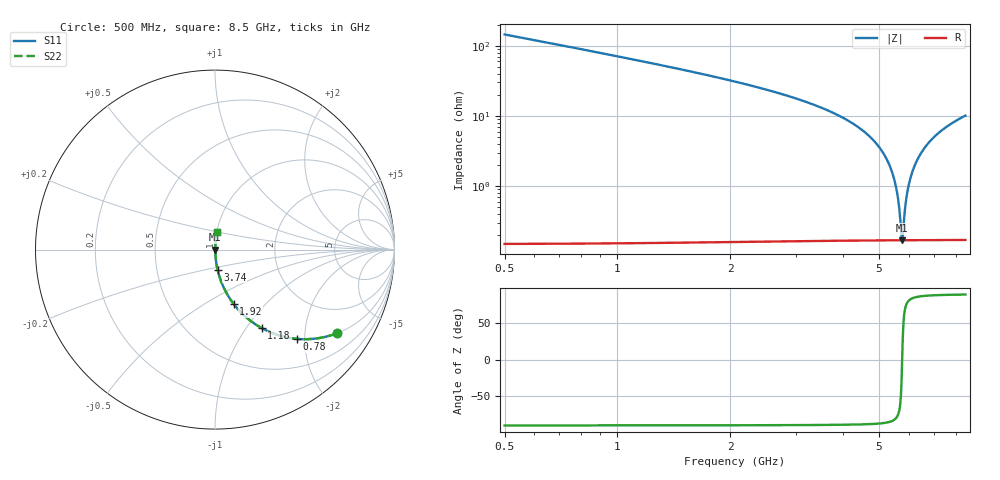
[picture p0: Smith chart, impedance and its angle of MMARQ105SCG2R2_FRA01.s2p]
! MMARQ105SCG2R2_FRA01  S-PARAMETER MODEL  ( General Type )
! Model Generated by TAIYO YUDEN Corporation (http://www.ty-top.com)
! Version 1.0
! TAIYO YUDEN Control No. 200326
! Copyright(c) 2020 TAIYO YUDEN CO.,LTD. All Rights Reserved.
! Product Description (link to TY-COMPAS)
! https://ds.yuden.co.jp/TYCOMPAS/or/detail?pn=MMARQ105SCG2R2BFRA01&u=M
! Products Name : Multilayer Ceramic Capacitors
! Characteristics :
!  Capacitance : 2.2 pF , Rated Voltage : 250V , TCC : CG / C0G
!  Case Size : 1.0 x 0.5 / 0.039 x 0.02 [mm/inch] , Thickness : 0.5 / 0.02 [mm/inch]
!  (Conditions: Temperature = 25 degC , DC Bias Current/Voltage = 0A / 0V)
! External Node Assignments :
!  1  o---| |---o  2
! GND o---------o GND
! Frequency Range : 500MHz  -  8.5GHz  [ 401 STEP ]
# MHz S RI R 50
! Freq[MHz].  S11 Real  S11 Imag  S21 Real  S21 Imag  S12 Real  S12 Imag  S22 Real  S22 Imag
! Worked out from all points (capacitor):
!   401 points, 500 MHz to 8.5 GHz, reference 50 ohm
!   read as one part in series: C = 2.18 pF near 540 MHz
!   lowest |Z| = 169 mohm at 5.76 GHz (marker M1)
!   series resonance near 5.762 GHz, so ESL is about 350 pH
!   S11 on the Smith chart (normalised r, x): 500 MHz: 1.00, -2.90; 780 MHz: 1.00, -1.84; 1.18 GHz: 1.00, -1.19; 1.92 GHz: 1.00, -0.68; 3.74 GHz: 1.00, -0.23; 8.5 GHz: 1.00, +0.20
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500  0.6773 -0.467  0.3227 0.467  0.3227 0.467  0.6773 -0.467
780  0.4579 -0.4974  0.5421 0.4974  0.5421 0.4974  0.4579 -0.4974
1180  0.2606 -0.4376  0.7394 0.4376  0.7394 0.4376  0.2606 -0.4376
1840  0.1137 -0.3153  0.8863 0.3153  0.8863 0.3153  0.1137 -0.3153
1920  0.1037 -0.3025  0.8963 0.3025  0.8963 0.3025  0.1037 -0.3025
3180  0.0264 -0.1552  0.9736 0.1552  0.9736 0.1552  0.0264 -0.1552
3740  0.0142 -0.1111  0.9858 0.1111  0.9858 0.1111  0.0142 -0.1111
4500  0.00564 -0.0628  0.9944 0.0628  0.9944 0.0628  0.00564 -0.0628
5020  0.0029 -0.0349  0.9971 0.0349  0.9971 0.0349  0.0029 -0.0349
5380  0.00199 -0.0173  0.998 0.0173  0.998 0.0173  0.00199 -0.0173
5580  0.00175 -0.0081  0.9982 0.0081  0.9982 0.0081  0.00175 -0.0081
5660  0.00171 -0.0045  0.9983 0.0045  0.9983 0.0045  0.00171 -0.0045
5720  0.00169 -0.00184  0.9983 0.00184  0.9983 0.00184  0.00169 -0.00184
5760  0.00169 -8.16e-05  0.9983 8.16e-05  0.9983 8.16e-05  0.00169 -8.16e-05
5800  0.00169 0.00167  0.9983 -0.00167  0.9983 -0.00167  0.00169 0.00167
5840  0.0017 0.0034  0.9983 -0.0034  0.9983 -0.0034  0.0017 0.0034
5900  0.00173 0.00598  0.9983 -0.00598  0.9983 -0.00598  0.00173 0.00598
5980  0.00178 0.00938  0.9982 -0.00938  0.9982 -0.00938  0.00178 0.00938
6240  0.0021 0.0201  0.9979 -0.0201  0.9979 -0.0201  0.0021 0.0201
6620  0.00293 0.0351  0.9971 -0.0351  0.9971 -0.0351  0.00293 0.0351
7180  0.00483 0.0558  0.9952 -0.0558  0.9952 -0.0558  0.00483 0.0558
8500  0.0117 0.0996  0.9883 -0.0996  0.9883 -0.0996  0.0117 0.0996
